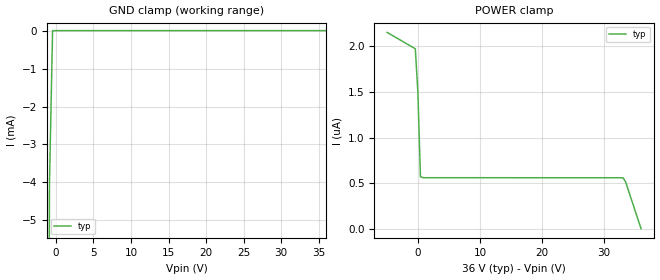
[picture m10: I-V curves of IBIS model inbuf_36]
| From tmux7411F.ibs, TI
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| inbuf_36
[Model]   inbuf_36
Model_type   Input
Vinl = 1.3
Vinh = 0.8
|   typ   min   max
C_comp   6.362683e-13   NA   NA
[Voltage Range]   36   NA   NA
[Temperature Range]   27   NA   NA
[Power Clamp Reference]   36   NA   NA
[GND Clamp Reference]   0   NA   NA
[GND Clamp]
|   Voltage   I(typ)   I(min)   I(max)
-5V       -369.9mA   NA         NA
-1.273V   -35.74mA   NA         NA
-858.6mV  -4.052mA   NA         NA
-444.4mV  -3.059uA   NA         NA
36V       1.411uA    NA         NA
[POWER Clamp]
|   Voltage   I(typ)   I(min)   I(max)
-5V       2.153uA    NA         NA
-444.4mV  1.974uA    NA         NA
-30.3mV   1.495uA    NA         NA
383.8mV   569.7nA    NA         NA
798mV     558.8nA    NA         NA
33.1V     557.4nA    NA         NA
33.52V    511.2nA    NA         NA
36V       -205.2pA   NA         NA
